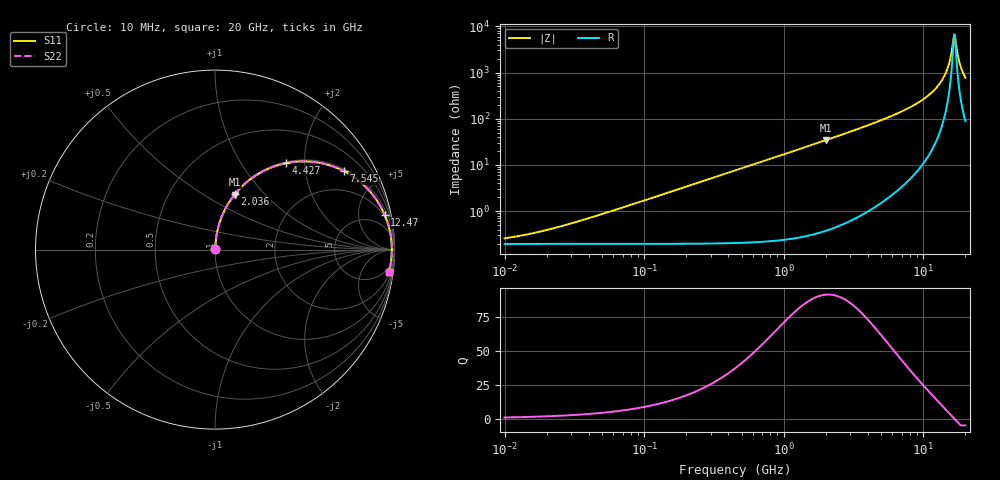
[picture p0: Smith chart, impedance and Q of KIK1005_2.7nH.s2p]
!version-3
!date-01.2023
!Series
# Hz S RI R 50
!Freq ReS11 ImS11 ReS21 ImS21 ReS12 ImS12 ReS22 ImS22
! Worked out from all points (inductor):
!   500 points, 10 MHz to 20 GHz, reference 50 ohm
!   read as one part in series: L = 2.7 nH near 34.87 MHz
!   highest Q = 91.4 at 2.005 GHz (marker M1), where L = 2.74 nH
!   self-resonance near 16.66 GHz
!   S11 on the Smith chart (normalised r, x): 10 MHz: 1.00, +0.00; 2.036 GHz: 1.01, +0.70; 4.427 GHz: 1.02, +1.62; 7.545 GHz: 1.08, +3.22; 12.47 GHz: 1.70, +9.54; 20 GHz: 3, -15
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1e7  0.00196 0.00169  0.998 -0.00169  0.998 -0.00169  0.00196 0.00169
1.783943e7  0.00197 0.00301  0.998 -0.00301  0.998 -0.00301  0.00197 0.00301
3.59488e7  0.00199 0.00607  0.998 -0.00607  0.998 -0.00607  0.00199 0.00607
1.272781e8  0.00243 0.0215  0.9976 -0.0215  0.9976 -0.0215  0.00243 0.0215
4.506326e8  0.00783 0.0757  0.9922 -0.0757  0.9922 -0.0757  0.00783 0.0757
1.595481e9  0.0719 0.2527  0.9281 -0.2527  0.9281 -0.2527  0.0719 0.2527
2.005031e9  0.1091 0.3063  0.8909 -0.3063  0.8909 -0.3063  0.1091 0.3063
2.035806e9  0.1121 0.3101  0.8879 -0.3101  0.8879 -0.3101  0.1121 0.3101
4.427068e9  0.3964 0.4818  0.6036 -0.4818  0.6036 -0.4818  0.3964 0.4818
5.648861e9  0.5387 0.4894  0.4613 -0.4894  0.4613 -0.4894  0.5387 0.4894
7.544864e9  0.7163 0.4382  0.2837 -0.4382  0.2837 -0.4382  0.7163 0.4382
1.007725e10  0.8686 0.3178  0.1314 -0.3178  0.1314 -0.3178  0.8686 0.3178
1.247257e10  0.9452 0.1941  0.0548 -0.1941  0.0548 -0.1941  0.9452 0.1941
1.36662e10  0.9662 0.135  0.0338 -0.135  0.0338 -0.135  0.9662 0.135
1.47477e10  0.9779 0.0841  0.0221 -0.0841  0.0221 -0.0841  0.9779 0.0841
1.543725e10  0.9823 0.0531  0.0177 -0.0531  0.0177 -0.0531  0.9823 0.0531
1.640708e10  0.9851 0.0114  0.0149 -0.0114  0.0149 -0.0114  0.9851 0.0114
1.665891e10  0.9852 0.000964  0.0148 -0.000964  0.0148 -0.000964  0.9852 0.000964
1.717422e10  0.9848 -0.0199  0.0152 0.0199  0.0152 0.0199  0.9848 -0.0199
1.797724e10  0.9826 -0.0512  0.0174 0.0512  0.0174 0.0512  0.9826 -0.0512
1.853333e10  0.98 -0.0719  0.02 0.0719  0.02 0.0719  0.98 -0.0719
2e10  0.9697 -0.1231  0.0303 0.1231  0.0303 0.1231  0.9697 -0.1231
